(* Logix 5000 Rung export; software revision 33.00 *)

TYPE Banner_IOL_Device :
STRUCT
   Initial_Global_Read : BOOL;
   Command : SINT;
   Data : Banner_IOL_Device_Index;
   Reset : BOOL;
END_STRUCT
END_TYPE

TYPE Banner_IOL_Device_Index :
STRUCT
   Index : Banner_IOL_Device_SubIndex[32];
END_STRUCT
END_TYPE

TYPE Banner_IOL_Device_SubIndex :
STRUCT
   Sub : DINT[34];
END_STRUCT
END_TYPE

TYPE Banner_IOL_Rules :
STRUCT
   Byte_Pos : SINT;   // Byte Position to read from or write data to.
   Multi : SINT;   // Determines if a multiple byte length index is being accessed. Use 2 for 2 bytes length, 3 for 3 byte length, etc..
   Sub_Index : SINT;
   Signed : SINT;   // 0=Unsigned, 1=Signed
END_STRUCT
END_TYPE

TYPE Banner_IOL_Rules_Array :
STRUCT
   Length : DINT;
   Settings : Banner_IOL_Rules_SettingsArray[32];
END_STRUCT
END_TYPE

TYPE Banner_IOL_Rules_SettingsArray :
STRUCT
   Index : DINT;
   Num_Op : INT;   // Number of Operations to read/write Index.
   Total_Bytes : INT;
   RW : SINT;   // 0 = Read Only, 1 = Write Only, 2 = Read or Write
   Rules : Banner_IOL_Rules[34];   // Sub Index Position in IODD.
END_STRUCT
END_TYPE

VAR_GLOBAL   (* controller tags *)
   R50CMDR_IOLM1_01 : Banner_IOL_Device;
        .DATA.INDEX[2]   // Direct Parameters 1
        .DATA.INDEX[2].SUB[1]   // Reserved
        .DATA.INDEX[2].SUB[2]   // Master Cycle Time
        .DATA.INDEX[2].SUB[3]   // Min Cycle Time
        .DATA.INDEX[2].SUB[4]   // M Sequence Capability
        .DATA.INDEX[2].SUB[5]   // IO-Link Version ID
        .DATA.INDEX[2].SUB[6]   // Process Data Input Length
        .DATA.INDEX[2].SUB[7]   // Process Data Output Length
        .DATA.INDEX[2].SUB[8]   // Vendor ID
        .DATA.INDEX[2].SUB[9]   // Device ID
        .DATA.INDEX[3]   // Standard Command
        .DATA.INDEX[3].SUB[1]   // Standard Command: 126=Locator Start, 127=Locator Stop, 129=Application Reset, 164=Reset All Metrics
        .DATA.INDEX[4]   // Serial Number
        .DATA.INDEX[4].SUB[1]   // SN1
        .DATA.INDEX[4].SUB[2]   // SN2
        .DATA.INDEX[4].SUB[3]   // SN3
        .DATA.INDEX[4].SUB[4]   // SN4
        .DATA.INDEX[4].SUB[5]   // SN5
        .DATA.INDEX[4].SUB[6]   // SN6
        .DATA.INDEX[4].SUB[7]   // SN7
        .DATA.INDEX[4].SUB[8]   // SN8
        .DATA.INDEX[4].SUB[9]   // SN9
        .DATA.INDEX[4].SUB[10]   // SN10
        .DATA.INDEX[4].SUB[11]   // SN11
        .DATA.INDEX[4].SUB[12]   // SN12
        .DATA.INDEX[4].SUB[13]   // SN13
        .DATA.INDEX[4].SUB[14]   // SN14
        .DATA.INDEX[4].SUB[15]   // SN15
        .DATA.INDEX[4].SUB[16]   // SN16
        .DATA.INDEX[5]   // All Time Run Time
        .DATA.INDEX[5].SUB[1]   // All Time Run Time
        .DATA.INDEX[6]   // Resettable Run Time
        .DATA.INDEX[6].SUB[1]   // Resettable Run Time
        .DATA.INDEX[7]   // Input Configuration
        .DATA.INDEX[7].SUB[1]   // Input Configuration: 0=BannerBus, 1=Discrete Input
        .DATA.INDEX[8]   // Port 1 Configuration
        .DATA.INDEX[8].SUB[1]   // Discrete 1 IO Selection: 0=NPN Input, 1=PNP Input, 2=NPN Output with Pull Up, 3=PNP Output with Pull Down, 4=NPN Output Push Pull, 5=PNPN Output Push Pull
        .DATA.INDEX[8].SUB[2]   // Discrete 1 Delay Mode: 0=Disabled, 1=On Off Delay, 2=On One-Shot, 3=Off One-Shot
        .DATA.INDEX[8].SUB[3]   // Discrete 1 Delay Timer 1
        .DATA.INDEX[8].SUB[4]   // Discrete 1 Delay Timer 2
        .DATA.INDEX[8].SUB[5]   // Discrete 2 IO Selection: 0=NPN Input, 1=PNP Input, 2=NPN Output with Pull Up, 3=PNP Output with Pull Down, 4=NPN Output Push Pull, 5=PNPN Output Push Pull
        .DATA.INDEX[8].SUB[6]   // Discrete 2 Delay Mode: 0=Disabled, 1=On Off Delay, 2=On One-Shot, 3=Off One-Shot
        .DATA.INDEX[8].SUB[7]   // Discrete 2 Delay Timer 1
        .DATA.INDEX[8].SUB[8]   // Discrete 2 Delay Timer 1
        .DATA.INDEX[9]   // Block Configuration
        .DATA.INDEX[9].SUB[1]   // Temperature High Setpoint
        .DATA.INDEX[9].SUB[2]   // Temperature Scale: 0=F, 1=C
        .DATA.INDEX[9].SUB[3]   // Undervoltage Alarm Setpoint
        .DATA.INDEX[9].SUB[4]   // Overvoltage Alarm Setpoint
        .DATA.INDEX[9].SUB[5]   // Analog Fix Speed Setting
        .DATA.INDEX[10]   // Motor Control Configuration
        .DATA.INDEX[10].SUB[1]   // Motor Power Enable: 0=Disabled, 1=Enabled
        .DATA.INDEX[10].SUB[2]   // Maximum Analog Setting
        .DATA.INDEX[10].SUB[3]   // Maximum Current Setting
        .DATA.INDEX[10].SUB[4]   // Current In-Rush Delay Setting
        .DATA.INDEX[10].SUB[5]   // Ramp On Delay
        .DATA.INDEX[10].SUB[6]   // Ramp Off Delay
        .DATA.INDEX[11]   // Monitoring
        .DATA.INDEX[11].SUB[1]   // Temperature F Reading
        .DATA.INDEX[11].SUB[2]   // Temperature C Reading
        .DATA.INDEX[11].SUB[3]   // Block Voltage Reading
        .DATA.INDEX[11].SUB[4]   // Current Reading
        .DATA.INDEX[12]   // Selectable Metric Reset
        .DATA.INDEX[12].SUB[1]   // Port 1 Discrete 1 Port 1 Discrete 2: see iodd file for information
        .DATA.INDEX[12].SUB[3]   // Port 1 Discrete 1 Reset Count
        .DATA.INDEX[12].SUB[4]   // Port 1 Discrete 2 Reset Count
        .DATA.INDEX[13]   // IO Metric Port 1
        .DATA.INDEX[13].SUB[1]   // Port 1 Discrete 1 Count
        .DATA.INDEX[13].SUB[2]   // Port 1 Discrete 1 Duration
        .DATA.INDEX[13].SUB[3]   // Port 1 Discrete 1 Events Per Minute
        .DATA.INDEX[13].SUB[4]   // Port 1 Discrete 1 Totalizer
        .DATA.INDEX[13].SUB[5]   // Port 1 Discrete 2 Count
        .DATA.INDEX[13].SUB[6]   // Port 1 Discrete 2 Duration
        .DATA.INDEX[13].SUB[7]   // Port 1 Discrete 2 Events Per Minute
        .DATA.INDEX[13].SUB[8]   // Port 1 Discrete 2 Totalizer
        .DATA.INDEX[14]   // Motor Run Time Configuration
        .DATA.INDEX[14].SUB[1]   // Motor Current ON Setting
        .DATA.INDEX[14].SUB[2]   // Resettable Motor Run Time
   R50CMDR_Rules : Banner_IOL_Rules_Array;
        .SETTINGS[2]   // Direct Parameters 1
        .SETTINGS[2].RULES[0]   // Reserved
        .SETTINGS[2].RULES[1]   // Master Cycle Time
        .SETTINGS[2].RULES[2]   // Min Cycle Time
        .SETTINGS[2].RULES[3]   // M-Sequence Capability
        .SETTINGS[2].RULES[4]   // IO-Link ID
        .SETTINGS[2].RULES[5]   // Process Data Input Length
        .SETTINGS[2].RULES[6]   // Process Data Output Length
        .SETTINGS[2].RULES[7]   // Vendor ID
        .SETTINGS[2].RULES[8]   // Device ID
        .SETTINGS[3]   // Standard Command
        .SETTINGS[3].RULES[0]   // Standard Command
        .SETTINGS[4]   // Serial Number
        .SETTINGS[4].RULES[0]   // SN1
        .SETTINGS[4].RULES[1]   // SN2
        .SETTINGS[4].RULES[2]   // SN3
        .SETTINGS[4].RULES[3]   // SN4
        .SETTINGS[4].RULES[4]   // SN5
        .SETTINGS[4].RULES[5]   // SN6
        .SETTINGS[4].RULES[6]   // SN7
        .SETTINGS[4].RULES[7]   // SN8
        .SETTINGS[4].RULES[8]   // SN9
        .SETTINGS[4].RULES[9]   // SN10
        .SETTINGS[4].RULES[10]   // SN11
        .SETTINGS[4].RULES[11]   // SN12
        .SETTINGS[4].RULES[12]   // SN13
        .SETTINGS[4].RULES[13]   // SN14
        .SETTINGS[4].RULES[14]   // SN15
        .SETTINGS[4].RULES[15]   // SN16
        .SETTINGS[5]   // All Time Run Time
        .SETTINGS[5].RULES[0]   // All Time Run Time
        .SETTINGS[6]   // Resettable Run Time
        .SETTINGS[6].RULES[0]   // Resettable Run Time
        .SETTINGS[7]   // Input Configuration
        .SETTINGS[7].RULES[0]   // Input Configuration
        .SETTINGS[8]   // Port 1 Configuration
        .SETTINGS[8].RULES[0]   // Discrete1 IO Selection
        .SETTINGS[8].RULES[1]   // Discrerte1 Delay Mode
        .SETTINGS[8].RULES[2]   // Discrete1 Delay Timer 1
        .SETTINGS[8].RULES[3]   // Discrete1 Delay Timer 2
        .SETTINGS[8].RULES[4]   // Discrete2 IO Selection
        .SETTINGS[8].RULES[5]   // Discrete2 Delay Mode
        .SETTINGS[8].RULES[6]   // Discrete2 Delay Timer 1
        .SETTINGS[8].RULES[7]   // Discrete2 Delay Timer 2
        .SETTINGS[9]   // Block Configuration
        .SETTINGS[9].RULES[0]   // Temperature High Setpoint
        .SETTINGS[9].RULES[1]   // Temperature Scale
        .SETTINGS[9].RULES[2]   // Undervoltage Alarm Setpoint
        .SETTINGS[9].RULES[3]   // Overvoltage Alarm Setpoint
        .SETTINGS[9].RULES[4]   // Analog Fix Speed Setting
        .SETTINGS[10]   // Motor Control Configuration
        .SETTINGS[10].RULES[0]   // Motor Power Enable
        .SETTINGS[10].RULES[1]   // Maximum Analog Setting
        .SETTINGS[10].RULES[2]   // Maximum Current Setting
        .SETTINGS[10].RULES[3]   // Current In-Rush Delay Setting
        .SETTINGS[10].RULES[4]   // Ramp On Delay
        .SETTINGS[10].RULES[5]   // Ramp Off Delay
        .SETTINGS[11]   // Monitoring
        .SETTINGS[11].RULES[0]   // Temperature F Reading
        .SETTINGS[11].RULES[1]   // Temperature C Reading
        .SETTINGS[11].RULES[2]   // Block Voltage Reading
        .SETTINGS[11].RULES[3]   // Current Reading
        .SETTINGS[12]   // Selectable Metric Reset
        .SETTINGS[12].RULES[0]   // Port 1 Discrete 1 / Port 1 Discrete 2
        .SETTINGS[12].RULES[1]   // Port 1 Discrete 1 Reset Count
        .SETTINGS[12].RULES[2]   // Port 1 Discrete 2 Reset Count
        .SETTINGS[13]   // IO Metric Port 1
        .SETTINGS[13].RULES[0]   // Port 1 Discrete 1 Count
        .SETTINGS[13].RULES[1]   // Port 1 Discrete 1 Duration
        .SETTINGS[13].RULES[2]   // Port 1 Discret 1 Events Per Minute
        .SETTINGS[13].RULES[3]   // Port 1 Discrete 1 Totalizer
        .SETTINGS[13].RULES[4]   // Port 1 Discrete 2 Count
        .SETTINGS[13].RULES[5]   // Port 1 Discrete 2 Duration
        .SETTINGS[13].RULES[6]   // Port 1 Discrete 2 Events Per Minute
        .SETTINGS[13].RULES[7]   // Port 1 Discrete 2 Totalizer
        .SETTINGS[14]   // Motor Run Time Configuration
        .SETTINGS[14].RULES[0]   // Motor Curret On Setting
        .SETTINGS[14].RULES[1]   // Resettable Motor Run Time
END_VAR

PROGRAM MainProgram

ROUTINE MainRoutine   (* ladder *)
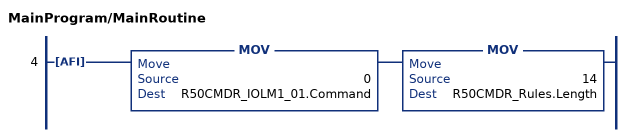
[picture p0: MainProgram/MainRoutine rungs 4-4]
   4: AFI()MOV(0,R50CMDR_IOLM1_01.Command)MOV(14,R50CMDR_Rules.Length);
END_ROUTINE
END_PROGRAM
